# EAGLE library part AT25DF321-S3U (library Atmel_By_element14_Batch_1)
Serial Flash Memory
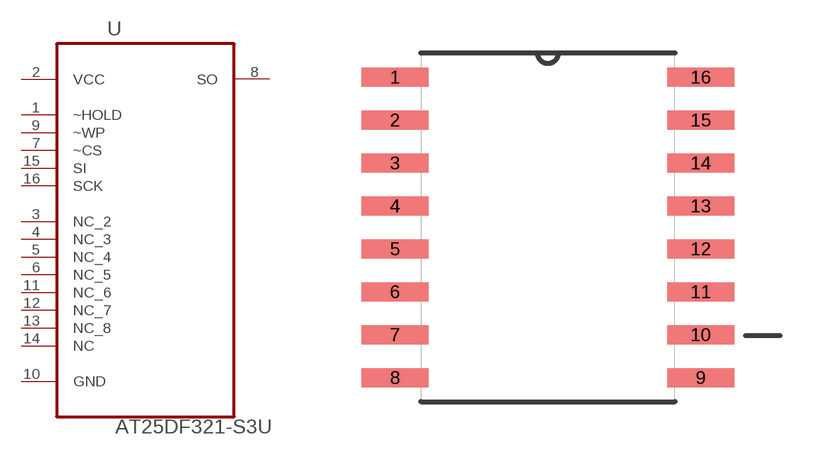
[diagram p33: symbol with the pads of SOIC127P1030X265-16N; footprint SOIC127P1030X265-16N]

Designator prefix U

## AT25DF321-S3U (MPN: AT25DF321-S3U; OC_FARNELL: 1636624; OC_NEWARK: 03P2053; PACKAGE: SOIC-16; SUPPLIER: Atmel)  [SOIC127P1030X265-16N]
1  ~HOLD  in
2  VCC  pwr
3  NC_2  nc
4  NC_3  nc
5  NC_4  nc
6  NC_5  nc
7  ~CS  in
8  SO  out
9  ~WP  in
10  GND  pas
11  NC_6  nc
12  NC_7  nc
13  NC_8  nc
14  NC  nc
15  SI  in
16  SCK  in

## Footprint SOIC127P1030X265-16N (pad centres in mm)
smd 1.981 x 0.559: 1 -4.521,4.445; 2 -4.521,3.175; 3 -4.521,1.905; 4 -4.521,0.635; 5 -4.521,-0.635; 6 -4.521,-1.905; 7 -4.521,-3.175; 8 -4.521,-4.445; 9 4.521,-4.445; 10 4.521,-3.175; 11 4.521,-1.905; 12 4.521,-0.635; 13 4.521,0.635; 14 4.521,1.905; 15 4.521,3.175; 16 4.521,4.445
